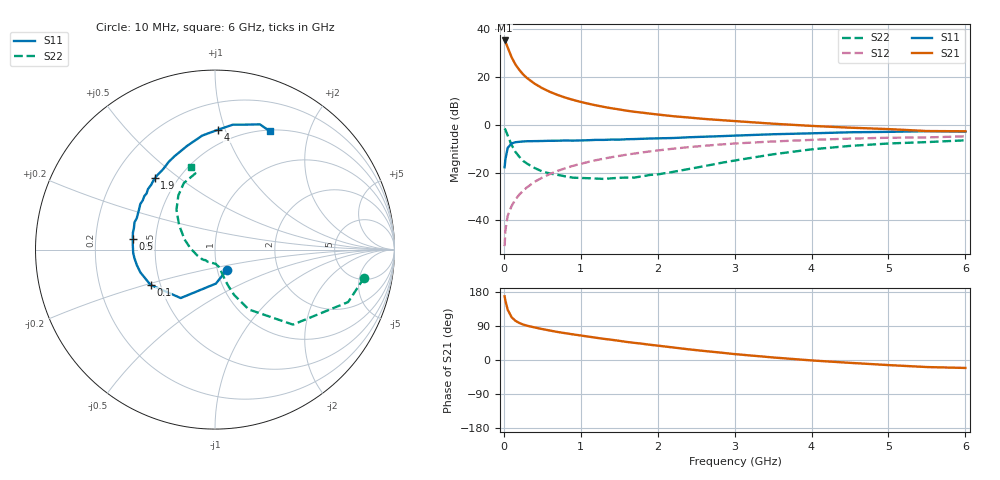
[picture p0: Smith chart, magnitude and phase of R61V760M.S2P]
! SIEMENS Small Signal Semiconductors
! BFR193
! Si NPN RF Bipolar Junction Transistor in SOT23
! VCE = 1.75 V  IC = 60 mA
! Common Emitter S-Parameters:  May  1996
# GHz  S  MA  R  50
!  f  S11  S21  S12  S22
! GHz  MAG  ANG  MAG  ANG  MAG  ANG  MAG  ANG
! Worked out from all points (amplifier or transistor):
!   36 points, 10 MHz to 6 GHz, reference 50 ohm
!   highest |S21| = 35.4 dB at 10 MHz (marker M1)
!   |S21| within 3 dB of that: start of sweep to 51.33 MHz
!   unconditionally stable (mu >= 1): 268.7 MHz to 2.212 GHz
!   at 250 MHz: K = 0.99, MSG = 24.4 dB, |S12| = -27.6 dB
!   at 1.4 GHz: K = 1.03, MAG = 9.2 dB, |S12| = -13.5 dB
!   at 6 GHz: K = 0.97, MSG = 1.0 dB, |S12| = -4.7 dB
!   S11 on the Smith chart (normalised r, x): 10 MHz: 1.12, -0.25; 100 MHz: 0.44, -0.21; 500 MHz: 0.37, +0.05; 1.9 GHz: 0.38, +0.41; 4 GHz: 0.39, +0.95; 6 GHz: 0.52, +1.44
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0.01  0.1305 -58.3  58.79 168.0  0.0029 76.2  0.8459 -10.6
0.02  0.1896 -88.6  55.53 156.8  0.0062 76.7  0.7974 -21.5
0.05  0.3307 -125.3  42.14 132.7  0.0125 69.5  0.6027 -43.9
0.1  0.4096 -151.3  26.37 113.2  0.02 68.3  0.3828 -60.6
0.15  0.4349 -163.1  18.57 103.5  0.0274 71.3  0.2747 -67.1
0.2  0.4439 -168.8  14.29 97.8  0.0347 73.3  0.2171 -69.8
0.25  0.4512 -173.8  11.48 93.7  0.0419 73.9  0.1782 -71.6
0.3  0.4562 -177.6  9.643 90.6  0.0493 74.6  0.1557 -72.7
0.4  0.4588 176.7  7.326 85.9  0.0646 75.0  0.1256 -74.2
0.5  0.4618 172.9  5.886 81.6  0.0792 74.7  0.1062 -75.6
0.6  0.4671 168.2  4.924 77.7  0.094 73.7  0.0964 -78.0
0.7  0.4675 165.1  4.25 73.9  0.1093 72.7  0.0901 -81.2
0.9  0.4697 158.2  3.35 67.6  0.1396 69.9  0.0788 -87.6
1.1  0.4791 151.9  2.783 61.7  0.1684 67.2  0.0767 -97.5
1.4  0.4941 142.8  2.236 53.4  0.2113 62.7  0.0764 -112.7
1.9  0.5202 130.2  1.729 40.2  0.2795 54.6  0.09 -143.9
2.2  0.5329 122.9  1.526 33.1  0.3183 49.6  0.1042 -161.7
3.5  0.6392 96.4  1.063 6.7  0.4512 28.2  0.2432 145.4
4  0.6684 88.5  0.956 -1.1  0.487 20.9  0.3086 134.1
4.5  0.7028 81.9  0.877 -7.5  0.5178 13.9  0.3643 124.1
5.5  0.7414 70.3  0.746 -18.6  0.5475 0.2  0.4379 104.5
6  0.7265 65.0  0.738 -21.0  0.5796 -3.8  0.4771 106.0
